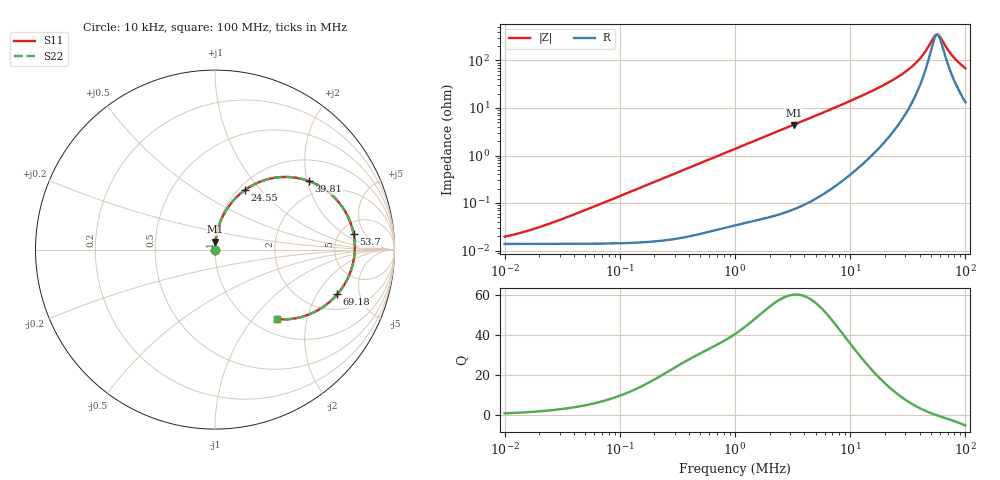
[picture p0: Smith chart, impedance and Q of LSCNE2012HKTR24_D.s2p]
! LSCNE2012HKTR24_D  S-PARAMETER MODEL  ( Standard Model )
! Model Generated by TAIYO YUDEN Corporation (http://www.ty-top.com)
! Version 1.0
! TAIYO YUDEN Control No. 210402
! Copyright(c) 2021 TAIYO YUDEN CO.,LTD. All Rights Reserved.
! Product Description (link to TY-COMPAS)
! https://ds.yuden.co.jp/TYCOMPAS/or/detail?pn=LSCNE2012HKTR24MD&u=M
! Products Name : Inductors
! Characteristics :
!  Inductance : 0.24 [uH] , SRF(min) : - [Hz] , DC Resistance(max) : 17 [mOhm]
!  Rated Current : Saturation  6.0 [A] (dL = 30 [%]), Temp Rise  4.8 [A] (dT = 40 [degC])
!  Case Size : 2.0 x 1.25 / 0.079 x 0.049 [mm/inch] , Thickness : 0.8 / 0.031 [mm/inch]
!  (Conditions: Temperature = 25 [degC] , DC Bias Current = 0 [A])
! External Node Assignments :
!  1  o---GGG---o  2
! GND o---------o GND
! Frequency Range : 10kHz  -  100MHz  [ 402 STEP ]
# MHz S RI R 50
! Freq[MHz].  S11 Real  S11 Imag  S21 Real  S21 Imag  S12 Real  S12 Imag  S22 Real  S22 Imag
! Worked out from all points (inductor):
!   401 points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, 10 kHz to 100 MHz, reference 50 ohm
!   read as one part in series: L = 222 nH near 30.2 kHz
!   highest Q = 60 at 3.236 MHz (marker M1), where L = 217 nH
!   self-resonance near 56.95 MHz
!   S11 on the Smith chart (normalised r, x): 10 kHz: 1.00, +0.00; 24.55 MHz: 1.07, +0.83; 39.81 MHz: 1.56, +2.05; 53.7 MHz: 6.68, +2.92; 69.18 MHz: 2.90, -3.05; 100 MHz: 1.26, -1.35
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0.01  0.000138 0.000139  0.9999 -0.000139  0.9999 -0.000139  0.000138 0.000139
0.019055  0.000138 0.000265  0.9999 -0.000265  0.9999 -0.000265  0.000138 0.000265
0.046774  0.000139 0.000651  0.9999 -0.000651  0.9999 -0.000651  0.000139 0.000651
0.218776  0.000168 0.00304  0.9998 -0.00304  0.9998 -0.00304  0.000168 0.00304
1  0.000527 0.0137  0.9995 -0.0137  0.9995 -0.0137  0.000527 0.0137
3.235937  0.00268 0.044  0.9973 -0.044  0.9973 -0.044  0.00268 0.044
4.677351  0.00519 0.0636  0.9948 -0.0636  0.9948 -0.0636  0.00519 0.0636
12.58925  0.0372 0.1726  0.9628 -0.1726  0.9628 -0.1726  0.0372 0.1726
16.98244  0.0713 0.2335  0.9287 -0.2335  0.9287 -0.2335  0.0713 0.2335
21.87762  0.1271 0.2992  0.8729 -0.2992  0.8729 -0.2992  0.1271 0.2992
24.54709  0.1671 0.3322  0.8329 -0.3322  0.8329 -0.3322  0.1671 0.3322
31.62278  0.3091 0.3958  0.6909 -0.3958  0.6909 -0.3958  0.3091 0.3958
35.48134  0.4063 0.4046  0.5937 -0.4046  0.5937 -0.4046  0.4063 0.4046
39.81072  0.523 0.3818  0.477 -0.3818  0.477 -0.3818  0.523 0.3818
45.70882  0.667 0.2892  0.333 -0.2892  0.333 -0.2892  0.667 0.2892
50.11872  0.7411 0.1832  0.2589 -0.1832  0.2589 -0.1832  0.7411 0.1832
53.70318  0.7725 0.0866  0.2275 -0.0866  0.2275 -0.0866  0.7725 0.0866
56.23413  0.7793 0.0185  0.2207 -0.0185  0.2207 -0.0185  0.7793 0.0185
58.88437  0.7744 -0.0491  0.2256 0.0491  0.2256 0.0491  0.7744 -0.0491
69.1831  0.6815 -0.249  0.3185 0.249  0.3185 0.249  0.6815 -0.249
81.28305  0.5305 -0.3585  0.4695 0.3585  0.4695 0.3585  0.5305 -0.3585
100  0.3474 -0.3879  0.6526 0.3879  0.6526 0.3879  0.3474 -0.3879
